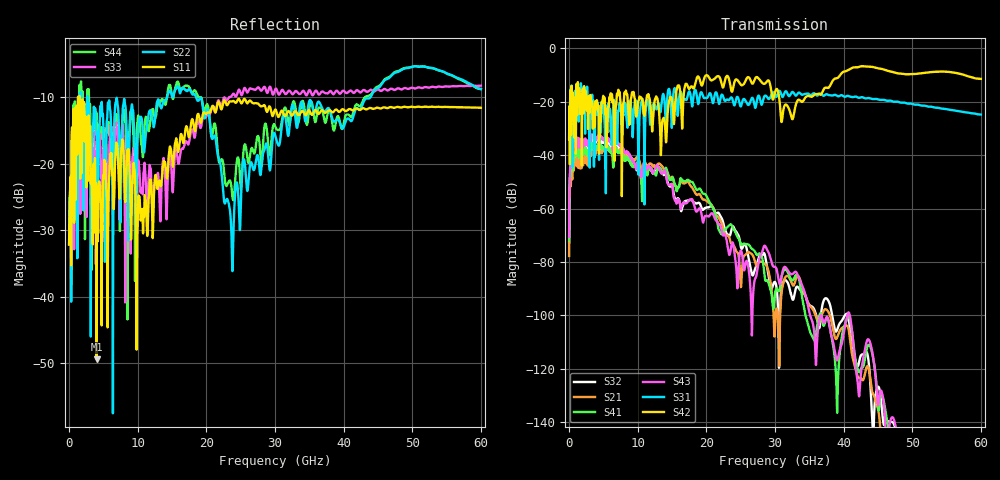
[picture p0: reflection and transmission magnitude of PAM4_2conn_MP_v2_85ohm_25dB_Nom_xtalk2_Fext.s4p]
! Info: Touchstone file created by Circ.  Input file=FAB50GbE_2conn_Midplane_Examax_Topo2_v2_85ohm_25dB_Nom.circ
# Hz S RI R 50
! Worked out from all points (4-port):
!   6000 points, 10 MHz to 60 GHz, reference 50 ohm
!   strongest paths, dB at 10 MHz, 15.01 GHz, 30.01 GHz, 45.01 GHz, 60 GHz:
!     S42: -34.0, -19.7, -16.3, -7.5, -11.4
!     S31: -33.9, -27.7, -17.5, -19.1, -24.8
!     S43: -70.6, -51.1, -81.8, -133.6, -181.0
!     S41: -71.8, -48.5, -91.7, -133.6, -196.8
!     S21: -77.7, -48.1, -103.6, -135.1, -188.2
!     S32: -72.6, -51.0, -87.5, -126.7, -169.6
!   lowest |S11| = -49.4 dB at 4.02 GHz (marker M1), VSWR 1.01, Z = 49.8 + j0.263 ohm
!   |S11| at or under -10 dB: start of sweep to 1.305 GHz; 1.323 GHz to 1.508 GHz (184.9 MHz wide, 13.1 % of centre); 1.54 GHz to end of sweep
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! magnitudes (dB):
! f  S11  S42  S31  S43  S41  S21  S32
! 10 MHz  -32.2  -34.0  -33.9  -70.6  -71.8  -77.7  -72.6
! 800 MHz  -13.9  -26.5  -18.5  -34.6  -37.8  -41.2  -36.4
! 4.02 GHz  -49.4  -19.5  -21.0  -33.4  -36.7  -37.9  -34.1
! 24.48 GHz  -10.6  -11.7  -18.2  -88.5  -70.4  -76.4  -69.1
! 32.51 GHz  -12.8  -26.5  -16.3  -84.5  -86.8  -88.3  -93.7
! 41.45 GHz  -12.0  -7.1  -18.2  -111.4  -111.0  -117.1  -113.8
! 60 GHz  -11.6  -11.4  -24.8  -181.0  -196.8  -188.2  -169.6
